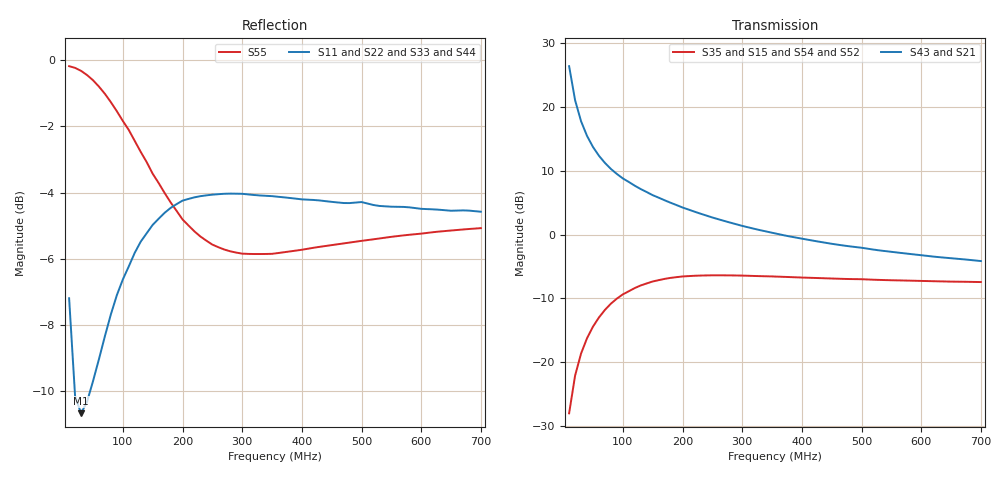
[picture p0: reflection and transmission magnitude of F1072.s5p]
! Date: Mon Aug 07 16:36:22 1995
!  POLYFET RF DEVICES
!  F1072 (Each Side)
!  S PARAMETERS
!  VDS=28V, IDQ=600mA
!AWR Design Environment (2053) Wed Feb 04 14:32:42 2004
!freq-unit  param-type  data-format  keyword  impedance-ohms
# MHz  S  MA  R  50
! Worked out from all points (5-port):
!   70 points, 10 MHz to 700 MHz, reference 50 ohm
!   strongest paths, dB at 10 MHz, 180 MHz, 360 MHz, 530 MHz, 700 MHz:
!     S43: 26.4, 5.0, 0.1, -2.5, -4.1
!     S21: 26.4, 5.0, 0.1, -2.5, -4.1
!     S35: -28.0, -6.8, -6.6, -7.1, -7.4
!     S15: -28.0, -6.8, -6.6, -7.1, -7.4
!     S54: -28.3, -7.0, -6.7, -7.1, -7.4
!     S52: -28.3, -7.0, -6.7, -7.1, -7.4
!   lowest |S11| = -10.7 dB at 30 MHz (marker M1), VSWR 1.83, Z = 48.2 - j30 ohm
!   |S11| at or under -10 dB: 19.51 MHz to 45.12 MHz (25.61 MHz wide, 79.2 % of centre)
